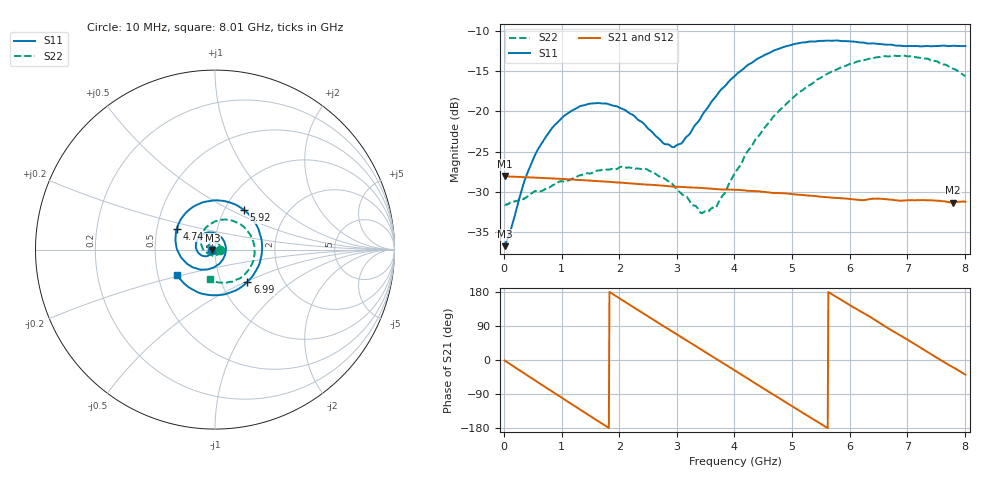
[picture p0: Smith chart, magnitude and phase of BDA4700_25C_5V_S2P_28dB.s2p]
!Agilent Technologies,E5071B,MY42404982,A.09.10
!Date: Mon Oct 20 13:40:39 2025
!Data & Calibration Information:
!Freq	S11:SOLT2(ON)	S21:SOLT2(ON)	S12:SOLT2(ON)	S22:SOLT2(ON)
# Hz S RI R 50
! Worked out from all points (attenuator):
!   801 points, 10 MHz to 8.01 GHz, reference 50 ohm
!   highest |S21| = -28.06 dB at 10 MHz (marker M1); lowest = -31.4 dB at 7.8 GHz (marker M2)
!   lowest |S11| = -36.8 dB at 10 MHz (marker M3), VSWR 1.03, Z = 48.6 - j0.132 ohm
!   |S11| at or under -10 dB: start of sweep to end of sweep
!   |S22| runs from -32.7 to -13.0 dB; largest |S21 - S12| = 0.00034
!   S11 on the Smith chart (normalised r, x): 10 MHz: 0.97, -0.00; 4.74 GHz: 0.63, +0.16; 5.92 GHz: 1.23, +0.59; 6.99 GHz: 1.33, -0.51; 8.01 GHz: 0.63, -0.19
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1e7  -0.0144 -0.00136  0.0395 -0.000811  0.0395 -0.000868  0.0262 -0.000823
3.7e8  -0.0265 -0.0275  0.0311 -0.0235  0.031 -0.0235  0.0216 -0.0191
5.8e8  -0.044 -0.0367  0.0205 -0.0327  0.0205 -0.0328  0.014 -0.0287
9.9e8  -0.0867 -0.0239  -0.00552 -0.0376  -0.00552 -0.0376  -0.014 -0.0338
1.35e9  -0.1071 0.0176  -0.0257 -0.027  -0.0258 -0.027  -0.036 -0.0178
1.97e9  -0.0554 0.0916  -0.0351 0.00875  -0.0351 0.00876  -0.0342 0.0276
2.68e9  0.051 0.045  -0.00481 0.0343  -0.00479 0.0343  0.0128 0.0375
2.92e9  0.0599 -0.000619  0.00876 0.0329  0.00876 0.0329  0.0245 0.0254
3.06e9  0.0554 -0.0295  0.0159 0.0299  0.0158 0.0299  0.0275 0.0149
3.44e9  0.00153 -0.0946  0.03 0.0146  0.03 0.0146  0.0187 -0.014
3.69e9  -0.0576 -0.1113  0.0328 0.0014  0.0328 0.00128  0.000673 -0.0256
4.01e9  -0.1409 -0.0885  0.0287 -0.0152  0.0287 -0.0152  -0.0322 -0.0258
4.39e9  -0.2115 0.00138  0.0139 -0.0286  0.014 -0.0287  -0.0685 0.00465
4.74e9  -0.2128 0.1173  -0.00387 -0.0308  -0.00378 -0.0308  -0.0792 0.0571
5.35e9  -0.0564 0.2662  -0.0269 -0.0127  -0.0269 -0.0128  -0.0158 0.1477
5.92e9  0.1608 0.222  -0.0254 0.0132  -0.0255 0.0132  0.1116 0.1555
6.28e9  0.2456 0.1032  -0.0145 0.0242  -0.0142 0.0242  0.1845 0.0999
6.68e9  0.2516 -0.066  0.00353 0.0281  0.00363 0.0281  0.2199 0.000765
6.99e9  0.1809 -0.1793  0.016 0.0229  0.0161 0.0229  0.2043 -0.0828
7.39e9  0.0243 -0.2529  0.0266 0.00845  0.0267 0.00843  0.1322 -0.1626
7.8e9  -0.151 -0.2069  0.0255 -0.00909  0.0256 -0.00914  0.0207 -0.1829
8.01e9  -0.2137 -0.1398  0.0213 -0.0172  0.0214 -0.0172  -0.0301 -0.1627
